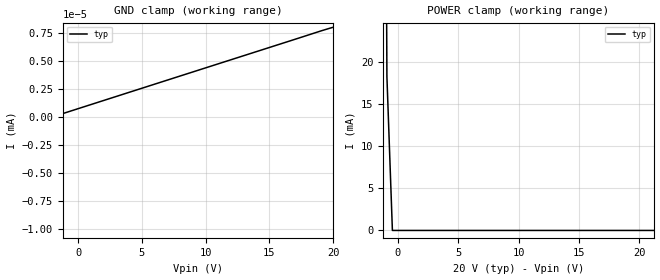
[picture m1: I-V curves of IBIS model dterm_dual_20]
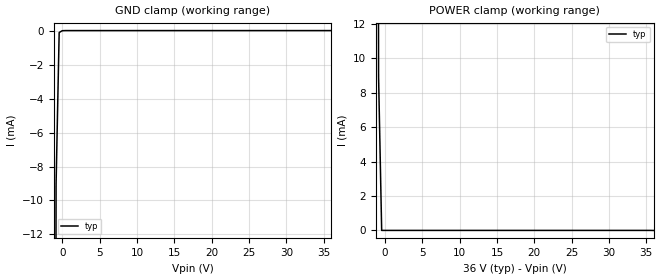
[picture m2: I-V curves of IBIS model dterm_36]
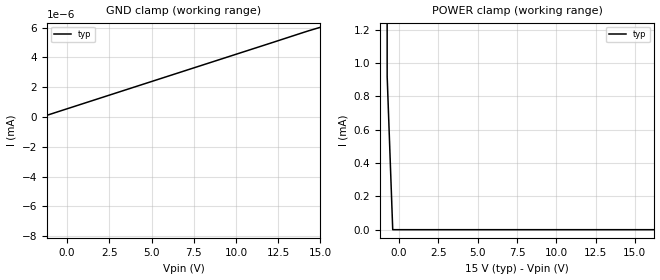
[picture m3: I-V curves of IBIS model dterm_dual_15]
|Texas Instruments Incorporated
|tmux7309f, 60-V Fault-Protected, Dual 4:1 Multiplexers with 1.8-V Logic
[IBIS Ver]   4.1
[File name]   tmux7309f.ibs
[Date]   12/09/21
[File Rev]   1.0
[Source]
| Texas Instruments Incorporated.
| ASC-INT-MPD
| 12500 TI Blvd
| Dallas, TX - 75243
[Notes]   Revision History:
| Rev 1.0: 12/09/21
| - Initial version of the model
| - Model generated from simulations in SPECTRE
| - C_comp although listed in numerical order of value are
|   obtained from varying PVT conditions. For PVT conditions for
|   each specific value refer the buffer description under
|   respective [Model]. IBIS model user is responsible for using
|   appropriate C_comp to simulate for Signal Integrity.
[Disclaimer]
| This model is designed as an aid for customers of Texas Instruments.
| TI and its licensors and suppliers make no warranties, either expressed
| or implied, with respect to this  model, including the warranties of
| merchantability or fitness for a particular purpose. The model is
| provided solely on an "as is" basis. The entire risk as to its quality
| and performance is with the customer.
| This model is subject to change without notice. Texas Instruments
| Incorporated is not responsible for updating this model.
[Copyright]
(C) Copyright 2021 Texas Instruments Incorporated.All rights reserved.
|  Component TMUX7309FPW 16-pin - PW package
|  Part # TMUX7309FPW
[Component]   TMUX7309FPW
[Manufacturer]  TI
[Package]
|   typ   min   max
R_pkg   0.0668   NA   NA
L_pkg   2.1992nH   NA   NA
C_pkg   0.2884pF   NA   NA
[Pin]   signal_name   model_name
   1   A0   inbuf
   2   EN   inbuf
   3   VSS   POWER
   4   S1A   sterm
   5   S2A   sterm
   6   S3A   sterm
   7   S4A   sterm
   8   DA   dterm
   9   DB   dterm
   10   S4B   sterm
   11   S3B   sterm
   12   S2B   sterm
   13   S1B   sterm
   14   VDD   POWER
   15   GND   GND
   16   A1   inbuf
[Series Switch Groups]
On 1 /
On 2 /
On 3 /
On 4 /
Off 1 2 3 4 /
[Series Pin Mapping]  pin_2 model_name function_table_group
   4   8   switch_dual_20   1
  13   9   switch_dual_20   1
   5   8   switch_dual_20   2
  12   9   switch_dual_20   2
   6   8   switch_dual_20   3
  11   9   switch_dual_20   3
   7   8   switch_dual_20   4
  10   9   switch_dual_20   4
|   4   8   switch_36   1
|  13   9   switch_36   1
|   5   8   switch_36   2
|  12   9   switch_36   2
|   6   8   switch_36   3
|  11   9   switch_36   3
|   7   8   switch_36   4
|  10   9   switch_36   4
|   4   8   switch_dual_15   1
|  13   9   switch_dual_15   1
|   5   8   switch_dual_15   2
|  12   9   switch_dual_15   2
|   6   8   switch_dual_15   3
|  11   9   switch_dual_15   3
|   7   8   switch_dual_15   4
|  10   9   switch_dual_15   4
|   4   8   switch_12   1
|  13   9   switch_12   1
|   5   8   switch_12   2
|  12   9   switch_12   2
|   6   8   switch_12   3
|  11   9   switch_12   3
|   7   8   switch_12   4
|  10   9   switch_12   4
|  Component TMUX7309FRRP 16-pin - RRP package
|  Part # TMUX7309FRRP
[Component]   TMUX7309FRRP
[Manufacturer]  TI
[Package]
|   typ   min   max
R_pkg   0.067   NA   NA
L_pkg   0.937nH   NA   NA
C_pkg   0.144pF   NA   NA
[Pin]   signal_name   model_name
   1   VSS   POWER
   2   S1A   sterm
   3   S2A   sterm
   4   S3A   sterm
   5   S4A   sterm
   6   DA   dterm
   7   DB   dterm
   8   S4B   sterm
   9   S3B   sterm
   10   S2B   sterm
   11   S1B   sterm
   12   VDD   POWER
   13   GND   GND
   14   A1   inbuf
   15   A0   inbuf
   16   EN   inbuf
[Series Switch Groups]
On 1 /
On 2 /
On 3 /
On 4 /
Off 1 2 3 4 /
[Series Pin Mapping]  pin_2 model_name function_table_group
   2   6   switch_dual_20   1
  11   7   switch_dual_20   1
   3   6   switch_dual_20   2
  10   7   switch_dual_20   2
   4   6   switch_dual_20   3
   9   7   switch_dual_20   3
   5   6   switch_dual_20   4
   8   7   switch_dual_20   4
|   2   6   switch_36   1
|  11   7   switch_36   1
|   3   6   switch_36   2
|  10   7   switch_36   2
|   4   6   switch_36   3
|   9   7   switch_36   3
|   5   6   switch_36   4
|   8   7   switch_36   4
|   2   6   switch_dual_15   1
|  11   7   switch_dual_15   1
|   3   6   switch_dual_15   2
|  10   7   switch_dual_15   2
|   4   6   switch_dual_15   3
|   9   7   switch_dual_15   3
|   5   6   switch_dual_15   4
|   8   7   switch_dual_15   4
|   2   6   switch_12   1
|  11   7   switch_12   1
|   3   6   switch_12   2
|  10   7   switch_12   2
|   4   6   switch_12   3
|   9   7   switch_12   3
|   5   6   switch_12   4
|   8   7   switch_12   4
[Model Selector] dterm
dterm_dual_20 Use for operation at +/-20V
dterm_36 Use for operation at 36V
dterm_dual_15 Use for operation at +/-15V
dterm_12 Use for operation at 12V
[Model Selector] sterm
sterm_dual_20 Use for operation at +/-20V
sterm_36 Use for operation at 36V
sterm_dual_15 Use for operation at +/-15V
sterm_12 Use for operation at 12V
[Model Selector] inbuf
inbuf_dual_20 Use for operation at +/-20V
inbuf_36 Use for operation at 36V
inbuf_dual_15 Use for operation at +/-15V
inbuf_12 Use for operation at 12V
| switch_dual_20
[Model]   switch_dual_20
Model_type   Series_switch
|   typ   min   max
C_comp   1.598234e-12   NA   NA
[Voltage Range]   20   NA   NA
[Power Clamp Reference]   20   NA   NA
[Temperature Range]   27   NA   NA
[On]
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[Off]
|   typ   min   max
[R Series]   10G   NA   NA
| switch_36
[Model]   switch_36
Model_type   Series_switch
|   typ   min   max
C_comp   1.598234e-12   NA   NA
[Voltage Range]   36   NA   NA
[Power Clamp Reference]   36   NA   NA
[Temperature Range]   27   NA   NA
[On]
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[Off]
|   typ   min   max
[R Series]   10G   NA   NA
| switch_dual_15
[Model]   switch_dual_15
Model_type   Series_switch
|   typ   min   max
C_comp   1.598234e-12   NA   NA
[Voltage Range]   15   NA   NA
[Power Clamp Reference]   15   NA   NA
[Temperature Range]   27   NA   NA
[On]
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[Off]
|   typ   min   max
[R Series]   10G   NA   NA
| switch_12
[Model]   switch_12
Model_type   Series_switch
|   typ   min   max
C_comp   2.533030e-12   NA   NA
[Voltage Range]   12   NA   NA
[Power Clamp Reference]   12   NA   NA
[Temperature Range]   27   NA   NA
[On]
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[Off]
|   typ   min   max
[R Series]   10G   NA   NA
| Models and submodels in the file (16): dterm_dual_20 (Terminator), dterm_36 (Terminator), dterm_dual_15 (Terminator), dterm_12 (Terminator), switch_dual_20 (Series_switch), switch_36 (Series_switch), switch_dual_15 (Series_switch), switch_12 (Series_switch), sterm_dual_20 (Terminator), sterm_36 (Terminator), sterm_dual_15 (Terminator), sterm_12 (Terminator), inbuf_dual_20 (Input), inbuf_36 (Input), inbuf_dual_15 (Input), inbuf_12 (Input)
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| dterm_dual_20
[Model]   dterm_dual_20
Model_type   Terminator
|   typ   min   max
C_comp   1.008417e-11   NA   NA
[Voltage Range]   20   NA   NA
[Temperature Range]   27   NA   NA
[Power Clamp Reference]   20   NA   NA
[GND Clamp Reference]   0   NA   NA
[GND Clamp]
|   Voltage   I(typ)   I(min)   I(max)
-25V      -1.414A    NA         NA
-20V      -5.041uA   NA         NA
-19.55V   -6.406nA   NA         NA
20V       8.043nA    NA         NA
[POWER Clamp]
|   Voltage   I(typ)   I(min)   I(max)
-5V       1.414A     NA         NA
-1.364V   155.3mA    NA         NA
-909.1mV  18.23mA    NA         NA
-454.5mV  68.57nA    NA         NA
40V       -5.036uA   NA         NA
| dterm_36
[Model]   dterm_36
Model_type   Terminator
|   typ   min   max
C_comp   1.008417e-11   NA   NA
[Voltage Range]   36   NA   NA
[Temperature Range]   27   NA   NA
[Power Clamp Reference]   36   NA   NA
[GND Clamp Reference]   0   NA   NA
[GND Clamp]
|   Voltage   I(typ)   I(min)   I(max)
-5V       -1.414A    NA         NA
-1.273V   -125.7mA   NA         NA
-858.6mV  -9.05mA    NA         NA
-444.4mV  -116uA     NA         NA
-30.3mV   -7.891uA   NA         NA
383.8mV   -5.778nA   NA         NA
36V       7.24nA     NA         NA
[POWER Clamp]
|   Voltage   I(typ)   I(min)   I(max)
-5V       1.414A     NA         NA
-1.273V   125.5mA    NA         NA
-858.6mV  8.924mA    NA         NA
-444.4mV  50.58nA    NA         NA
36V       -4.424uA   NA         NA
| dterm_dual_15
[Model]   dterm_dual_15
Model_type   Terminator
|   typ   min   max
C_comp   1.008417e-11   NA   NA
[Voltage Range]   15   NA   NA
[Temperature Range]   27   NA   NA
[Power Clamp Reference]   15   NA   NA
[GND Clamp Reference]   0   NA   NA
[GND Clamp]
|   Voltage   I(typ)   I(min)   I(max)
-20V      -1.414A    NA         NA
-15.05V   -11.62uA   NA         NA
-14.7V    -4.947nA   NA         NA
-14.34V   -4.692nA   NA         NA
15V       6.031nA    NA         NA
[POWER Clamp]
|   Voltage   I(typ)   I(min)   I(max)
-5V       1.414A     NA         NA
-1.111V   74.09mA    NA         NA
-757.6mV  919.6uA    NA         NA
-404mV    15.19nA    NA         NA
29.65V    -857.9pA   NA         NA
30V       -4.915uA   NA         NA
